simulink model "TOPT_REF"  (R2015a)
settings: Solver=ode3  StartTime=0.0  StopTime=trun  FixedStep=1e-8  MaxStep=dt/100  RelTol=1e-12
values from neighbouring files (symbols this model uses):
  A = sys.a    [fig2_plot_FTO_REF.m]    (also in fig4_ptosref_udot.m; fig6_7_plotdata_REF.m = ptosParams.A)
  B = sys.b    [fig2_plot_FTO_REF.m]    (also in fig4_ptosref_udot.m; fig6_7_plotdata_REF.m = ptosParams.B)
  c = bo/w^2    [fig2_plot_FTO_REF.m]    (also in fig4_ptosref_udot.m; fig6_7_plotdata_REF.m = ptosParams.c; fig1_motivate_ptos.m = 4.59233914625; f_ptos.m = ptosParams.c)
  cbar_min = ptosParams.cbar_min    [fig6_7_plotdata_REF.m]    (also in fptosref.m)
  cbar_plus = ptosParams.cbar_plus    [fig6_7_plotdata_REF.m]    (also in fptosref.m)
  Ts = ptosParams.Ts    [fig6_7_plotdata_REF.m]
  umax = 1 - x1r/c    [fig2_plot_FTO_REF.m]    (also in fig4_ptosref_udot.m; fig6_7_plotdata_REF.m = ptosParams.umax)
  umin = -1 - x1r/c    [fig2_plot_FTO_REF.m]    (also in fig4_ptosref_udot.m; fig6_7_plotdata_REF.m = ptosParams.umin)
  w = sqrt(-A(2,1))    [fig2_plot_FTO_REF.m]    (also in fig4_ptosref_udot.m; fig6_7_plotdata_REF.m = ptosParams.w; fig1_motivate_ptos.m = 1994.91133503; fptosref.m = ptosParams.w)
  X0 = [y(1), vhat(1)]'    [fig6_7_plotdata_REF.m]
  x1r = -0.4*c    [fig2_plot_FTO_REF.m]    (also in fig4_ptosref_udot.m = -0.5*c; fig6_7_plotdata_REF.m = ptosParams.x1r)
  x1Tol = c/100    [fig4_ptosref_udot.m]    (also in fig6_7_plotdata_REF.m = 0.005*c)
  x2Tol = (bo/w)/100    [fig4_ptosref_udot.m]    (also in fig6_7_plotdata_REF.m = .005*(bo/w))
  xell_plus = ptosParams.xell_plus    [fig6_7_plotdata_REF.m]    (also in fptosref.m; ptosDampRef.m = wp*e2(1))
libraries: simulink x2

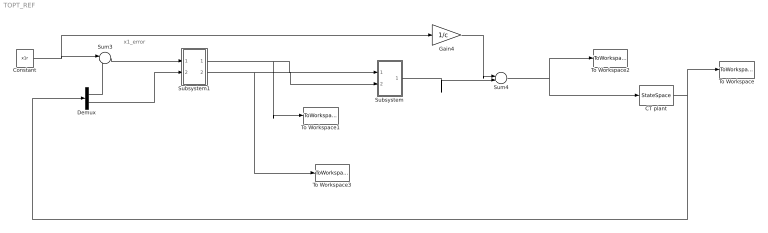
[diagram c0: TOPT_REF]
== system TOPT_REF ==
  note: x1_error
  CT plant : StateSpace  A=A  B=B  C=eye(2)  D=[0;0]  X0=X0
  Constant : Constant  Value=x1r
  Demux : Demux  Outputs=2
  Gain4 : Gain  Gain=1/c
  Subsystem : Subsystem
  Subsystem1 : Subsystem
  Sum3 : Sum  Inputs=|-+
  Sum4 : Sum  Inputs=|++
  To Workspace : ToWorkspace  VariableName=xplant_to  SaveFormat=Timeseries  SampleTime=Ts
  To Workspace1 : ToWorkspace  VariableName=x11  SaveFormat=Timeseries  SampleTime=Ts
  To Workspace2 : ToWorkspace  VariableName=uto  SaveFormat=Timeseries  SampleTime=Ts
  To Workspace3 : ToWorkspace  VariableName=x22  SaveFormat=Timeseries  SampleTime=Ts
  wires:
  CT plant/1 -> Demux/1, To Workspace/1
  Sum4/1 -> CT plant/1, To Workspace2/1
  Constant/1 -> Gain4/1, Sum3/1
  Gain4/1 -> Sum4/1
  Subsystem/1(u(k)) -> Sum4/2
  Demux/1 -> Sum3/2
  Demux/2 -> Subsystem1/2(In2)
  Sum3/1 -> Subsystem1/1(In1)
  Subsystem1/1(Out1) -> To Workspace1/1, Subsystem/1(x1e)
  Subsystem1/2(Out2) -> To Workspace3/1, Subsystem/2(x2)

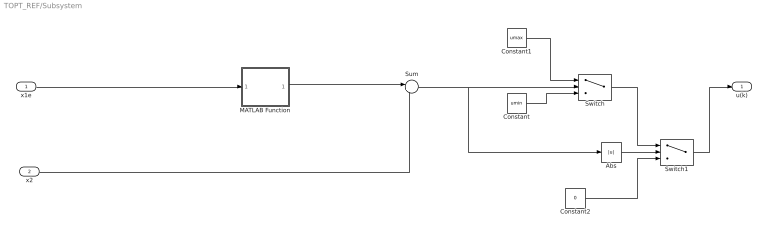
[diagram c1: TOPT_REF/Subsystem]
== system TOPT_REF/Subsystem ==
  x1e : Inport
  x2 : Inport  Port=2
  Abs : Abs
  Constant : Constant  Value=umin
  Constant1 : Constant  Value=umax
  Constant2 : Constant  Value=0
  MATLAB Function : MATLAB Function  TreatAsAtomicUnit=on
  Sum : Sum  Inputs=|+-
  Switch : Switch  Criteria=u2 > Threshold
  Switch1 : Switch  Criteria=u2 > Threshold
  u(k) : Outport
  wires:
  MATLAB Function/1(fto) -> Sum/1
  x2/1 -> Sum/2
  x1e/1 -> MATLAB Function/1(x1e)
  Constant/1 -> Switch/3
  Constant1/1 -> Switch/1
  Sum/1 -> Abs/1, Switch/2
  Abs/1 -> Switch1/2
  Switch/1 -> Switch1/1
  Constant2/1 -> Switch1/3
  Switch1/1 -> u(k)/1

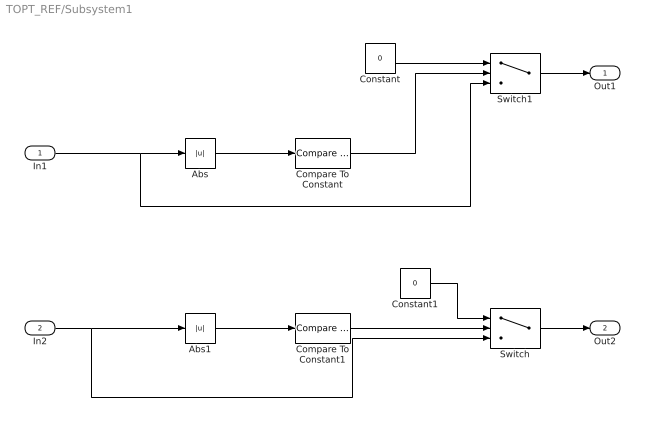
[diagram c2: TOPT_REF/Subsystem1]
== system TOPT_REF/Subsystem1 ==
  In1 : Inport
  In2 : Inport  Port=2
  Abs : Abs
  Abs1 : Abs
  Compare To Constant : simulink/Logic and Bit Operations/Compare To Constant  relop=<=  const=x1Tol  OutDataTypeStr=boolean
  Compare To Constant1 : simulink/Logic and Bit Operations/Compare To Constant  relop=<=  const=x2Tol  OutDataTypeStr=boolean
  Constant : Constant  Value=0
  Constant1 : Constant  Value=0
  Switch : Switch  Criteria=u2 > Threshold
  Switch1 : Switch  Criteria=u2 > Threshold
  Out1 : Outport
  Out2 : Outport  Port=2
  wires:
  Switch/1 -> Out2/1
  Abs/1 -> Compare To Constant/1
  In1/1 -> Switch1/3, Abs/1
  Abs1/1 -> Compare To Constant1/1
  In2/1 -> Switch/3, Abs1/1
  Switch1/1 -> Out1/1
  Compare To Constant/1 -> Switch1/2
  Constant/1 -> Switch1/1
  Compare To Constant1/1 -> Switch/2
  Constant1/1 -> Switch/1

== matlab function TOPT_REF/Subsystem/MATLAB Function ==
function fto = fcn(x1e, xell_plus, cbar_min, cbar_plus, w)
%#codegen


if (x1e < 0)
   fto =  w*sqrt(2*cbar_min*abs(x1e) -x1e.^2);
elseif(x1e > 0 )
    fto   = -w*sqrt(2*cbar_plus*x1e -x1e.^2);
else 
    fto = 0;
end







end
